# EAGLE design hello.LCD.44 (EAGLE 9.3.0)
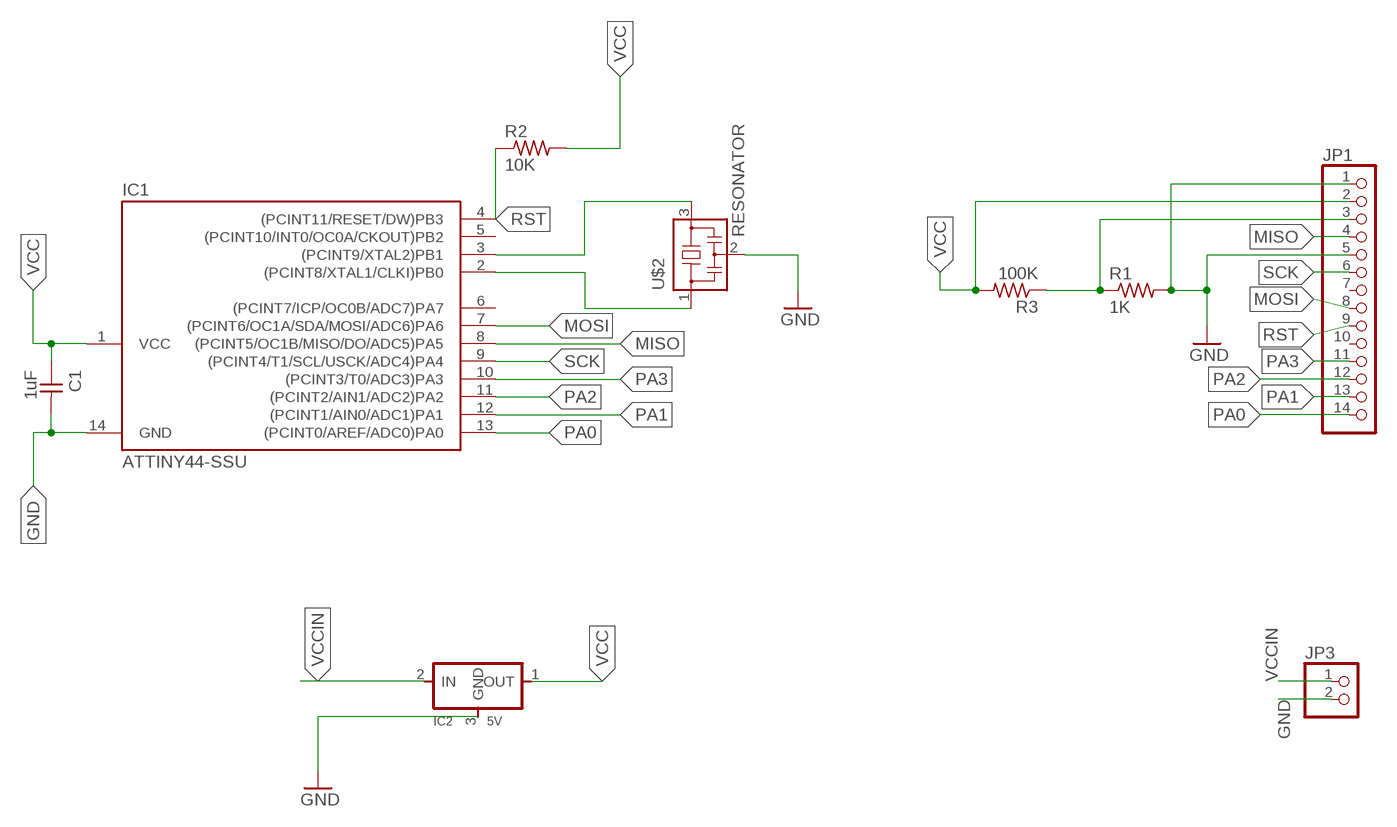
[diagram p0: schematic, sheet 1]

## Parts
C1  1uF  CAP-UNPOLARIZEDFAB  [C1206FAB]
IC1  ATTINY44-SSU  [SOIC14]
IC2  5V  REGULATORSOT23  [SOT23]
JP1  PINHD-1X14  [1X14]
JP3  PINHD-1X2/90  [1X02/90]
R1  1K  RES-US1206FAB  [R1206FAB]
R2  10K  RES-US1206FAB  [R1206FAB]
R3  100K  RES-US1206FAB  [R1206FAB]
U$2  RESONATOR  [EFOBM]

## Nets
GND: C1.2 IC1.14(GND) IC2.3(GND) JP1.1 JP1.5 JP3.2 R1.2 U$2.2
MISO: IC1.8((PCINT5/OC1B/MISO/DO/ADC5)PA5) JP1.4
MOSI: IC1.7((PCINT6/OC1A/SDA/MOSI/ADC6)PA6) JP1.8
N$1: IC1.3((PCINT9/XTAL2)PB1) U$2.3
N$2: IC1.2((PCINT8/XTAL1/CLKI)PB0) U$2.1
N$5: JP1.3 R1.1 R3.1
PA0: IC1.13((PCINT0/AREF/ADC0)PA0) JP1.14
PA1: IC1.12((PCINT1/AIN0/ADC1)PA1) JP1.13
PA2: IC1.11((PCINT2/AIN1/ADC2)PA2) JP1.12
PA3: IC1.10((PCINT3/T0/ADC3)PA3) JP1.11
RST: IC1.4((PCINT11/RESET/DW)PB3) JP1.9 R2.1
SCK: IC1.9((PCINT4/T1/SCL/USCK/ADC4)PA4) JP1.6
VCC: C1.1 IC1.1(VCC) IC2.1(OUT) JP1.2 R2.2 R3.2
VCCIN: IC2.2(IN) JP3.1
Unconnected: IC1.5((PCINT10/INT0/OC0A/CKOUT)PB2) IC1.6((PCINT7/ICP/OC0B/ADC7)PA7) JP1.7 JP1.10

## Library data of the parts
C1 = fab:CAP-UNPOLARIZED
IC1 = fab:ATTINY44
IC2 = fab:REGULATOR
JP1 = pinhead:PINHD-1X14: PIN HEADER
JP3 = pinhead:PINHD-1X2: PIN HEADER
R1-R3 = fab:RES-US: Resistor (US Symbol)
U$2 = fab:RESONATOR

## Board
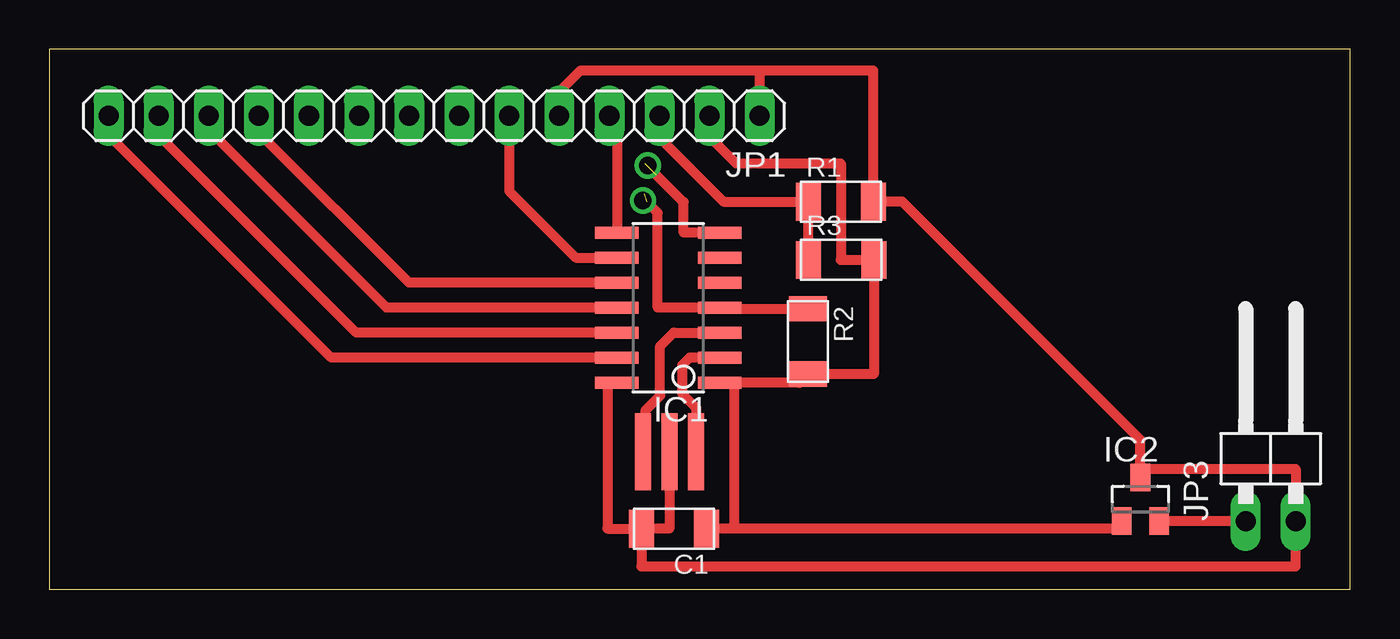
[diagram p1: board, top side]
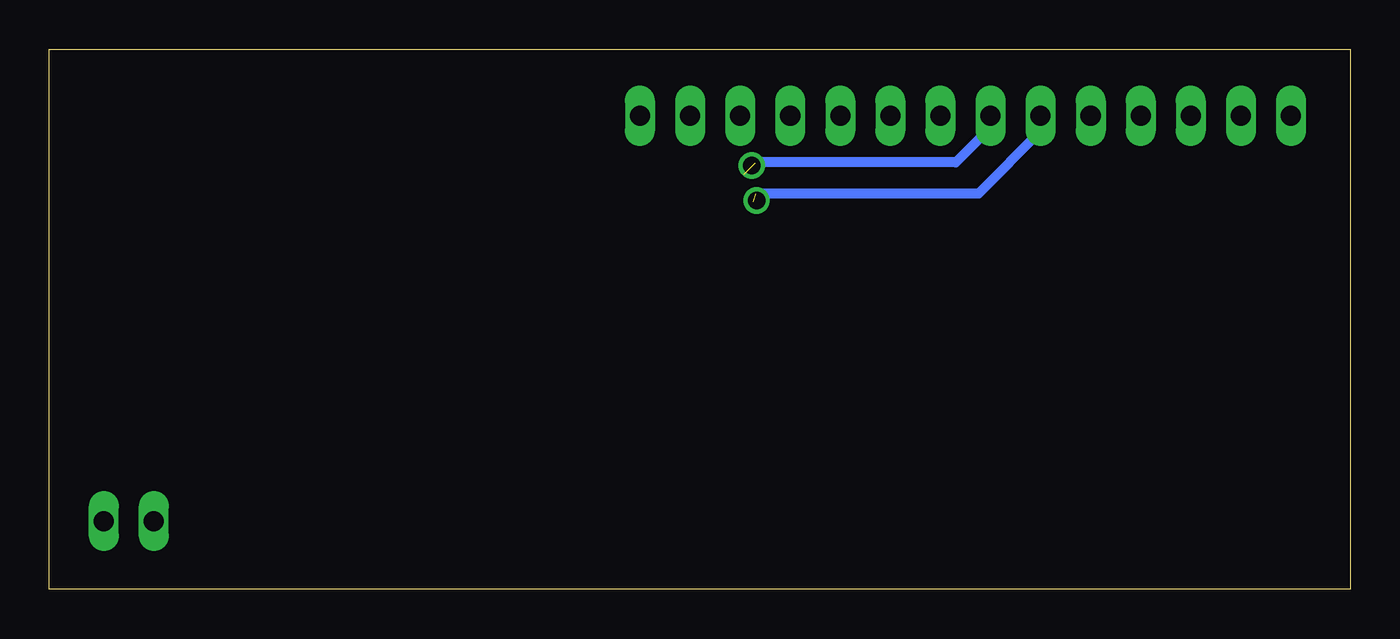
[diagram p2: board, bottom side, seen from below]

Size 66 x 27.39 mm. Coordinates in mm from the lower left corner, seen from the top.
Outline: 0,0 66,0 66,27.39 0,27.39 0,0
Copper layers (1*16): Top 0.035mm / dielectric 1.5mm / Bottom 0.035mm
Design rules "default": minimum track width 6mil, minimum drill 0.35mm, track to track 6mil, track to pad 6mil, pad to pad 6mil, via to via 6mil, smd to smd 6mil, copper to edge 40mil, drill to drill 6mil, minimum pad ring 10mil, minimum via ring 8mil, stop-mask expansion 4mil, vias tented up to drill 0mil, thermal gap 10mil

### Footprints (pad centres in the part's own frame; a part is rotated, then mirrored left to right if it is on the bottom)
C1206FAB = smd 1.27 x 1.905: 1 -1.651,0; 2 1.651,0
SOIC14 = smd 0.61 x 2.21: 1 -3.81,-2.603; 2 -2.54,-2.603; 3 -1.27,-2.603; 4 0,-2.603; 5 1.27,-2.603; 6 2.54,-2.603; 7 3.81,-2.603; 8 3.81,2.603; 9 2.54,2.603; 10 1.27,2.603; 11 0,2.603; 12 -1.27,2.603; 13 -2.54,2.603; 14 -3.81,2.603
SOT23 = smd 1 x 1.4: 1 -0.95,-1.1; 2 0.95,-1.1; 3 0,1.1
1X14 = drill 1.016 long: 1 -16.51,0; 2 -13.97,0; 3 -11.43,0; 4 -8.89,0; 5 -6.35,0; 6 -3.81,0; 7 -1.27,0; 8 1.27,0; 9 3.81,0; 10 6.35,0; 11 8.89,0; 12 11.43,0; 13 13.97,0; 14 16.51,0
1X02/90 = drill 1.016 long: 1 -1.27,-3.81; 2 1.27,-3.81
R1206FAB = smd 1.27 x 1.905: 1 -1.651,0; 2 1.651,0
EFOBM = smd 0.8 x 3.9: 1 -1.35,0; 2 0,0; 3 1.35,0

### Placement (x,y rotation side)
C1  31.69,3.07 180 top
IC1  31.4,14.28 90 top
IC2  55.36,4.58 0 top
JP1  19.52,24.02 180 top
JP3  61.97,7.27 0 top
R1  40.16,19.66 0 top
R2  38.49,12.57 270 top
R3  40.18,16.71 0 top
U$2  31.47,6.97 180 top

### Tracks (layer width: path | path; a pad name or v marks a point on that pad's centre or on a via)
GND
  Top 0.508: IC1.14 28.32,10.47 28.32,3.07 C1.2 | JP1.5 25.87,25.23 26.96,26.32 36.03,26.32 | 36.03,26.32 JP1.1 | 36.03,26.32 41.81,26.32 R1.2 43.28,19.66 55.36,7.58 IC2.3 55.77,6.09 63.24,6.09 JP3.2 63.24,1.17 30.04,1.17 C1.2 | U$2.2 31.47,3.07 C1.2
MISO
  Top 0.508: JP1.4 28.8,23.63 IC1.8
MOSI  (1 unrouted)
  Top 0.508: IC1.7 32.18,18.09 32.18,19.63 30.78,21.04
  Bottom 0.508: JP1.8 18.25,23.41 20.01,21.65 30.16,21.65 30.2,21.61
N$1
  Top 0.508: U$2.3 30.26,7.11 30.26,9.09 31,9.83 31,12.33 31.68,13.02 IC1.3
N$2
  Top 0.508: IC1.2 34,11.76 32.49,11.76 32.1,11.37 32.1,9.92 32.82,9.21 U$2.1
N$3  (via drill 0.89 pad 0.76)
  other vias: 30.12,19.72
N$4  (via drill 0.89 pad 0.76)
  other vias: 30.36,21.49
N$5
  Top 0.508: R3.1 38.51,16.72 R1.1 34.2,19.66 30.95,22.91 JP1.3
PA0
  Top 0.508: IC1.13 14.3,11.74 3.01,23.04 JP1.14
PA1
  Top 0.508: IC1.12 15.57,13.02 5.55,23.04 JP1.13
PA2
  Top 0.508: IC1.11 17.1,14.29 8.09,23.3 JP1.12
PA3
  Top 0.508: IC1.10 18.24,15.55 10.63,23.17 JP1.11
RST  (1 unrouted)
  Top 0.508: R2.1 34.07,14.22 IC1.4 30.88,14.29 30.86,14.3 30.86,19.09 30.29,19.66
  Bottom 0.508: JP1.9 15.71,23.22 18.86,20.07 30.17,20.07
SCK
  Top 0.508: JP1.6 23.33,20.19 26.7,16.82 IC1.9
VCC
  Top 0.508: JP1.2 33.49,22.96 34.85,21.6 40.16,21.6 40.16,16.71 R3.2 41.83,10.92 R2.2 38.05,10.47 IC1.1 34.73,10.47 34.73,3.07 C1.1 54.01,3.07 IC2.1
VCCIN
  Top 0.508: IC2.2 60.68,3.48 JP3.1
